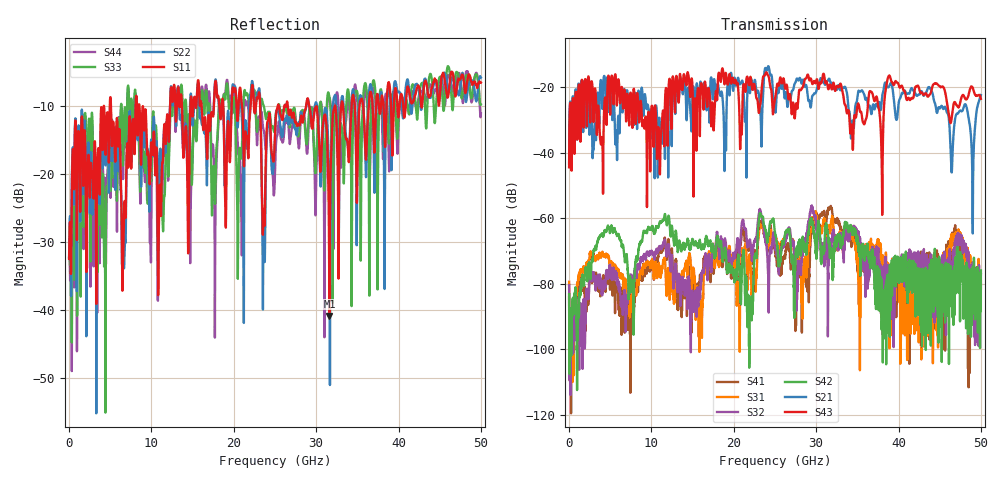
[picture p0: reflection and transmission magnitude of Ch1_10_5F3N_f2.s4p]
!Agilent Technologies,N5247A,US51170199,A.09.90.13
!Agilent N5247A: A.09.90.13
!Date: Wednesday, December 09, 2015 09:33:45
!Correction: S11(Full 4 Port(1,2,3,4))
!S12(Full 4 Port(1,2,3,4))
!S13(Full 4 Port(1,2,3,4))
!S14(Full 4 Port(1,2,3,4))
!S21(Full 4 Port(1,2,3,4))
!S22(Full 4 Port(1,2,3,4))
!S23(Full 4 Port(1,2,3,4))
!S24(Full 4 Port(1,2,3,4))
!S31(Full 4 Port(1,2,3,4))
!S32(Full 4 Port(1,2,3,4))
!S33(Full 4 Port(1,2,3,4))
!S34(Full 4 Port(1,2,3,4))
!S41(Full 4 Port(1,2,3,4))
!S42(Full 4 Port(1,2,3,4))
!S43(Full 4 Port(1,2,3,4))
!S44(Full 4 Port(1,2,3,4))
!S4P File: Measurements: <S11,S12,S13,S14>,
!<S21,S22,S23,S24>,
!<S31,S32,S33,S34>,
!<S41,S42,S43,S44>:
# Hz S  dB  R 50
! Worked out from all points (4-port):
!   3201 points, 10 MHz to 50 GHz, reference 50 ohm
!   strongest paths, dB at 10 MHz, 12.51 GHz, 25 GHz, 37.5 GHz, 50 GHz:
!     S43: -44.4, -19.7, -23.6, -25.5, -23.5
!     S21: -43.3, -27.2, -25.8, -26.1, -22.4
!     S42: -83.2, -62.5, -64.4, -76.5, -75.9
!     S32: -80.4, -71.9, -69.2, -71.0, -77.0
!     S31: -79.4, -76.0, -65.8, -67.8, -79.2
!     S41: -84.1, -69.9, -70.2, -73.8, -81.3
!   lowest |S11| = -40.9 dB at 31.61 GHz (marker M1), VSWR 1.02, Z = 50.7 - j0.555 ohm
!   |S11| at or under -10 dB: start of sweep to 4.949 GHz; 8.54 GHz to 12.26 GHz (3.72 GHz wide, 35.8 % of centre); 29.15 GHz to 32.29 GHz (3.133 GHz wide, 10.2 % of centre)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
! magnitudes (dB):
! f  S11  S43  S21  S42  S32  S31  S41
! 10 MHz  -32.5  -44.4  -43.3  -83.2  -80.4  -79.4  -84.1
! 12.59 GHz  -9.3  -16.7  -18.8  -64.3  -76.3  -80.1  -74.3
! 23.65 GHz  -25.3  -16.5  -17.5  -61.9  -63.4  -64.5  -64.9
! 28.94 GHz  -9.0  -16.2  -21.9  -66.5  -63.2  -73.1  -82.3
! 31.61 GHz  -40.9  -19.4  -17.5  -68.8  -67.9  -63.0  -56.7
! 49 GHz  -6.8  -20.1  -60.4  -80.9  -77.8  -82.2  -73.6
! 50 GHz  -6.6  -23.5  -22.4  -75.9  -77.0  -79.2  -81.3
